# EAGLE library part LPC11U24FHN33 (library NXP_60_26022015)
32-bit ARM Cortex-M0 microcontroller; up to 32 kB flash; up to 10 kB SRAM and 4 kB EEPROM; USB device; USART The LPC11U2x are an ARM Cortex-M0 based, low-cost 32-bit MCU family, designed for 8/16-bit microcontroller applications, offering performance, low power, simple instruction set and memory addressing together with reduced code size compared to existing 8/16-bit architectures. The LPC11U2x operate at CPU frequencies of up to 50 MHz. Equipped with a highly flexible and configurable Full-Speed USB 2.0 device controller, the LPC11U2x brings unparalleled design flexibility and seamless integration to today’s demanding connectivity solutions. The peripheral complement of the LPC11U2x includes up to 32 kB of flash memory, up to 10 kB of SRAM data memory and 4 kB EEPROM, one Fast-mode Plus I 2 C-bus interface, one RS-485/EIA-485 USART with support for synchronous mode and smart card interface, two SSP interfaces, four general-purpose counter/timers, a 10-bit ADC (Analog-to-Digital Converter), and up to 54 general-purpose I/O pins. AAL Eindhoven MK
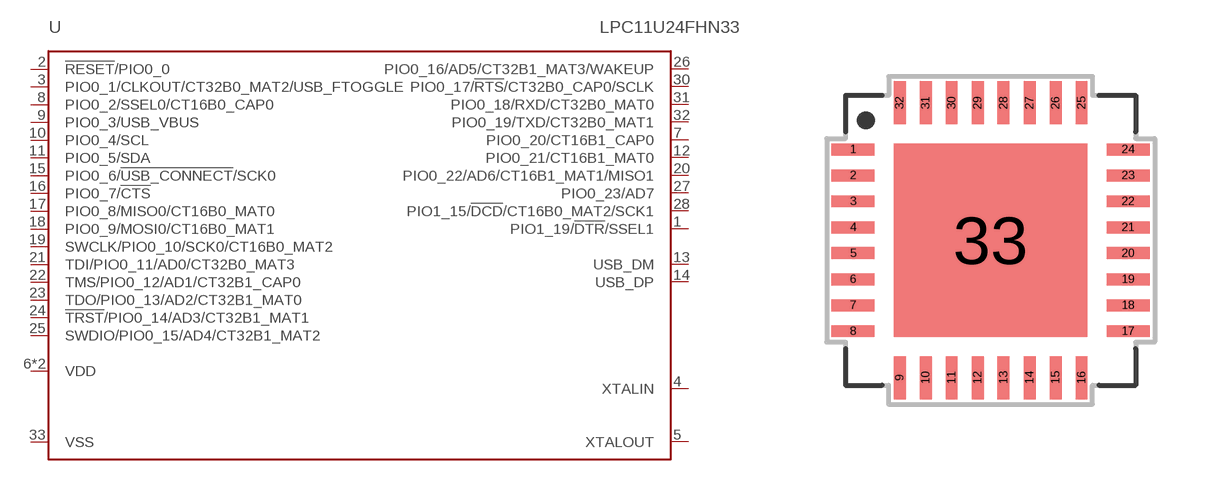
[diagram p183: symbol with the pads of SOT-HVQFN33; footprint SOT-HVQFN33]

Designator prefix U

## LPC11U24FHN33/401 (EEPROM: 4kB; FLASH: 32kB; GPIO: 26; SRAM: 8kB; USB_SRAM: 2kB)  [SOT-HVQFN33]
1  PIO1_19/!DTR!/SSEL1
2  !RESET!/PIO0_0
3  PIO0_1/CLKOUT/CT32B0_MAT2/USB_FTOGGLE
4  XTALIN  in
5  XTALOUT  out
6  VDD  pwr
7  PIO0_20/CT16B1_CAP0
8  PIO0_2/SSEL0/CT16B0_CAP0
9  PIO0_3/USB_VBUS
10  PIO0_4/SCL
11  PIO0_5/SDA
12  PIO0_21/CT16B1_MAT0
13  USB_DM
14  USB_DP
15  PIO0_6/!USB_CONNECT!/SCK0
16  PIO0_7/!CTS!
17  PIO0_8/MISO0/CT16B0_MAT0
18  PIO0_9/MOSI0/CT16B0_MAT1
19  SWCLK/PIO0_10/SCK0/CT16B0_MAT2
20  PIO0_22/AD6/CT16B1_MAT1/MISO1
21  TDI/PIO0_11/AD0/CT32B0_MAT3
22  TMS/PIO0_12/AD1/CT32B1_CAP0
23  TDO/PIO0_13/AD2/CT32B1_MAT0
24  !TRST!/PIO0_14/AD3/CT32B1_MAT1
25  SWDIO/PIO0_15/AD4/CT32B1_MAT2
26  PIO0_16/AD5/CT32B1_MAT3/WAKEUP
27  PIO0_23/AD7
28  PIO1_15/!DCD!/CT16B0_MAT2/SCK1
29  VDD  pwr
30  PIO0_17/!RTS!/CT32B0_CAP0/SCLK
31  PIO0_18/RXD/CT32B0_MAT0
32  PIO0_19/TXD/CT32B0_MAT1
33  VSS  pwr

## Footprint SOT-HVQFN33 (pad centres in mm)
SOTxxx HVQFN33: plastic thermal enhanced very thin quad flat package; no leads; 33 terminals; body 7 x 7 x 0.85 mm JEDEC: --- IEC: --- Package according LPC111x datasheet
smd 1.075 x 0.3: 1 -3.438,2.275; 2 -3.438,1.625; 3 -3.438,0.975; 4 -3.438,0.325; 5 -3.438,-0.325; 6 -3.438,-0.975; 7 -3.438,-1.625; 8 -3.438,-2.275; 17 3.438,-2.275; 18 3.438,-1.625; 19 3.438,-0.975; 20 3.438,-0.325; 21 3.438,0.325; 22 3.438,0.975; 23 3.438,1.625; 24 3.438,2.275
smd 0.3 x 1.075: 9 -2.275,-3.438; 10 -1.625,-3.438; 11 -0.975,-3.438; 12 -0.325,-3.438; 13 0.325,-3.438; 14 0.975,-3.438; 15 1.625,-3.438; 16 2.275,-3.438; 25 2.275,3.438; 26 1.625,3.438; 27 0.975,3.438; 28 0.325,3.438; 29 -0.325,3.438; 30 -0.975,3.438; 31 -1.625,3.438; 32 -2.275,3.438
smd 4.85 x 4.85: 33 0,0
